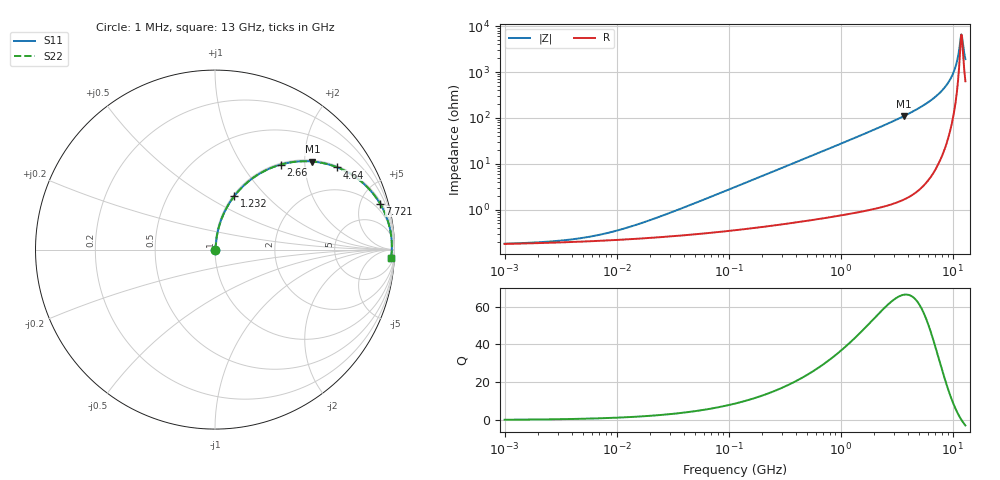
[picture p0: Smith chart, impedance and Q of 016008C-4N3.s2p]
# MHz S MA R 50
!Freq  MagS11  AngS11  MagS21  AngS21  MagS12  AngS12  MagS22  AngS22
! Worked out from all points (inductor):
!   801 points, 1 MHz to 13 GHz, reference 50 ohm
!   read as one part in series: L = 4.3 nH near 28.87 MHz
!   highest Q = 66.2 at 3.662 GHz (marker M1), where L = 4.74 nH
!   self-resonance near 11.97 GHz
!   S11 on the Smith chart (normalised r, x): 1 MHz: 1.00, +0.00; 1.232 GHz: 1.02, +0.67; 2.66 GHz: 1.02, +1.51; 4.64 GHz: 1.05, +2.95; 7.721 GHz: 1.24, +7.12; 13 GHz: 14, -36
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1  0.001799 8.6  0.9982 -0.0  0.9982 -0.0  0.001799 8.6
2.488668  0.002 19.6  0.9981 -0.0  0.9981 -0.0  0.002 19.6
4.887486  0.002394 33.3  0.998 -0.1  0.998 -0.1  0.002394 33.3
10.18395  0.003503 51.4  0.9978 -0.2  0.9978 -0.2  0.003503 51.4
23.60634  0.006828 68.4  0.9975 -0.4  0.9975 -0.4  0.006828 68.4
114.0175  0.03089 81.7  0.996 -1.8  0.996 -1.8  0.03089 81.7
557.2591  0.1485 79.2  0.9831 -8.5  0.9831 -8.5  0.1485 79.2
1231.969  0.3166 70.2  0.9409 -18.5  0.9409 -18.5  0.3166 70.2
1820.959  0.4464 62.4  0.8862 -26.5  0.8862 -26.5  0.4464 62.4
2659.854  0.5983 52.3  0.7915 -36.7  0.7915 -36.7  0.5983 52.3
2691.536  0.6033 52.0  0.7877 -37.1  0.7877 -37.1  0.6033 52.0
3661.874  0.7318 42.1  0.6706 -47.0  0.6706 -47.0  0.7318 42.1
4640.364  0.8217 33.9  0.5572 -55.2  0.5572 -55.2  0.8217 33.9
6165.529  0.908 23.6  0.401 -65.2  0.401 -65.2  0.908 23.6
7721.052  0.9546 15.5  0.268 -72.6  0.268 -72.6  0.9546 15.5
9005.919  0.9745 10.1  0.1749 -76.6  0.1749 -76.6  0.9745 10.1
10018.67  0.9824 6.3  0.1103 -77.7  0.1103 -77.7  0.9824 6.3
10756.34  0.9851 3.8  0.0676 -75.4  0.0676 -75.4  0.9851 3.8
11548.33  0.9856 1.3  0.02711 -57.4  0.02711 -57.4  0.9856 1.3
11825.08  0.9854 0.5  0.01703 -30.5  0.01703 -30.5  0.9854 0.5
12252.68  0.9845 -0.7  0.02002 38.9  0.02002 38.9  0.9845 -0.7
13000  0.9819 -2.8  0.05143 68.0  0.05143 68.0  0.9819 -2.8
